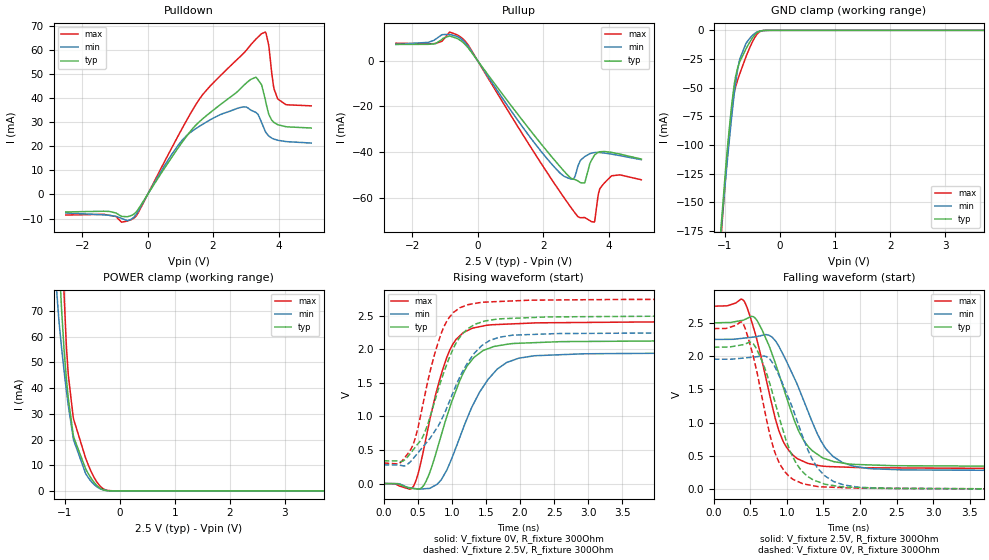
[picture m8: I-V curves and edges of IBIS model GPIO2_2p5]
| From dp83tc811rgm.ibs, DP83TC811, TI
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|   GPIO2_2p5 Model
[Model]   GPIO2_2p5
Model_type   I/O
Polarity   Non-Inverting
Enable   Active-Low
Vinl = 0.7
Vinh = 1.7
Vmeas = 1.25
Vref = 0
Cref = 2pF
Rref = 100000
|   typ   min   max
C_comp   3.2185pF   3.0315pF   3.3393pF
| Where Nom  PVT is Nominal Process, 2.5V, 27C
|   Fast PVT is Strong Process,  2.75V, -40C
|   Slow PVT is Weak Process,   2.25V, 125C
[Voltage Range]   2.5   2.25   2.75
|Junction Temperature
[Temperature Range]   27   125   -40
[Pullup Reference]   2.5   2.25   2.75
[Pulldown Reference]   0   0   0
[Power Clamp Reference]   2.5   2.25   2.75
[GND Clamp Reference]   0   0   0
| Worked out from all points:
|   slope of the pulldown table from 0 to 0.375 V, typ, clamps not added: 47.1 ohm
|   slope of the pullup table from 0 to 0.375 V, typ, clamps not added: 51.4 ohm
|   GND clamp passes 1 mA (typ) near -0.38 V on its own axis
|   POWER clamp passes 1 mA (typ) near -0.35 V on its own axis
|   falling waveform, V_fixture 2.5V, R_fixture 300Ohm: 20-80 % time 426ps typ, 473ps min, 334ps max; typ from 2.5 V to 0.339 V
|   rising waveform, V_fixture 0V, R_fixture 300Ohm: 20-80 % time 439ps typ, 535ps min, 364ps max; typ from 0 V to 2.13 V
|   rising waveform, V_fixture 2.5V, R_fixture 300Ohm: 20-80 % time 442ps typ, 590ps min, 359ps max; typ from 0.339 V to 2.5 V
|   falling waveform, V_fixture 0V, R_fixture 300Ohm: 20-80 % time 377ps typ, 428ps min, 307ps max; typ from 2.13 V to 0 V
[Pulldown]
|   Voltage   I(typ)   I(min)   I(max)
-2.5V     -7.255mA   -7.666mA   -8.536mA
-407.5mV  -8.044mA   -9.291mA   -9.718mA
747.5mV   15.65mA    16.84mA    19.61mA
1.34V     26.78mA    26.11mA    34.31mA
2.9V      44.79mA    36.31mA    58.19mA
3.312V    48.7mA     34.06mA    64.56mA
3.485V    45.46mA    29.83mA    66.8mA
3.62V     37.78mA    25.65mA    66.86mA
3.71V     33.06mA    24.21mA    61.1mA
3.845V    30.12mA    23.09mA    45.22mA
3.98V     28.98mA    22.52mA    39.66mA
5V        27.61mA    21.36mA    36.81mA
[GND Clamp]
|   Voltage   I(typ)   I(min)   I(max)
-2.5V     -1.255A    -1.134A    -1.35A
-1.067V   -171.4mA   -175.1mA   -180.1mA
-985mV    -120.8mA   -129.8mA   -127.2mA
-962.5mV  -108.2mA   -118.1mA   -113.7mA
-880mV    -67.32mA   -77.6mA    -70.77mA
-842.5mV  -52.25mA   -61.1mA    -57.64mA
-805mV    -40.55mA   -46.45mA   -49.4mA
-730mV    -27.57mA   -25.3mA    -38.07mA
-617.5mV  -16.29mA   -11.63mA   -23.27mA
-407.5mV  -1.86mA    -1.33mA    -3.018mA
-197.5mV  -14.99uA   -21.02uA   -19.14uA
5V        0A         0A         0A
[Pullup]
|   Voltage   I(typ)   I(min)   I(max)
-2.5V     7.194mA    7.203mA    7.713mA
-1.278V   7.641mA    9.595mA    7.627mA
-850mV    10.89mA    11.57mA    12.6mA
-437.5mV  7.916mA    8.747mA    9.422mA
2.397V    -44.38mA   -47.43mA   -54.94mA
2.915V    -51.88mA   -51.81mA   -65.59mA
3.065V    -52.69mA   -46.03mA   -68.29mA
3.268V    -53.51mA   -41.98mA   -68.7mA
3.56V     -41.53mA   -40.23mA   -70.73mA
3.695V    -40mA      -40.19mA   -57.87mA
4.1V      -40.17mA   -40.92mA   -50.36mA
5V        -43.06mA   -43.34mA   -52.15mA
[POWER Clamp]
|   Voltage   I(typ)   I(min)   I(max)
-2.5V     1.378A     1.128A     1.575A
-1.173V   138.2mA    86.25mA    204.3mA
-1.105V   95.25mA    67.15mA    145.5mA
-1.075V   79.94mA    60.23mA    121.4mA
-1.06V    73.26mA    56.99mA    110.2mA
-1.008V   54.58mA    46.52mA    75.98mA
-970mV    44.54mA    39.67mA    57.97mA
-932.5mV  36.21mA    33.3mA     45.26mA
-842.5mV  21.82mA    20.63mA    28.66mA
-617.5mV  8.611mA    6.772mA    12.78mA
-355mV    1.092mA    848.1uA    1.9mA
5V        0A         0A         0A
[Ramp]
R_load = 300
|   typ   min   max
dV/dt_r   1.27951/4.3828e-10   1.17145/5.33755e-10   1.44729/3.6279e-10
dV/dt_f   1.29582/4.22384e-10   1.1823/4.69132e-10   1.46485/3.31231e-10
[Falling Waveform]
V_fixture = 2.5V
V_fixture_min = 2.25V
V_fixture_max = 2.75V
R_fixture = 300Ohm
C_fixture = 0F
|   Time   V(typ)   V(min)   V(max)
0s        2.498V     2.249V     2.749V
419.9ps   2.546V     2.27V      2.815V
574.2ps   2.559V     2.289V     2.31V
800.6ps   2.02V      2.281V     1.245V
1.034ns   1.249V     1.828V     571mV
1.233ns   727mV      1.321V     413.3mV
1.464ns   488.1mV    726.4mV    349.6mV
1.761ns   392.8mV    400.5mV    332.7mV
2.586ns   351.9mV    289.5mV    318.7mV
20ns      338.8mV    278.7mV    307.4mV
[Rising Waveform]
V_fixture = 0V
V_fixture_min = 0V
V_fixture_max = 0V
R_fixture = 300Ohm
C_fixture = 0F
|   Time   V(typ)   V(min)   V(max)
0s        95.73uV    179.9uV    141.9uV
408.7ps   -70.99mV   -66mV      -75.15mV
583.6ps   -32.26mV   -77.9mV    491.2mV
769.5ps   459.9mV    -18.73mV   1.353V
972.7ps   1.141V     311.6mV    1.995V
1.221ns   1.745V     963.2mV    2.275V
1.506ns   2V         1.514V     2.357V
1.979ns   2.09V      1.867V     2.383V
2.927ns   2.117V     1.933V     2.4V
20ns      2.133V     1.953V     2.412V
[Rising Waveform]
V_fixture = 2.5V
V_fixture_min = 2.25V
V_fixture_max = 2.75V
R_fixture = 300Ohm
C_fixture = 0F
|   Time   V(typ)   V(min)   V(max)
0s        338.8mV    278.7mV    307.4mV
229ps     330.3mV    275.2mV    299.7mV
419.9ps   485.7mV    357.3mV    550.9mV
605.9ps   770.4mV    582.9mV    1.326V
791.5ps   1.37V      844.8mV    2.078V
933ps     1.797V     1.145V     2.434V
1.143ns   2.217V     1.643V     2.629V
1.414ns   2.398V     2.029V     2.697V
2.542ns   2.483V     2.234V     2.735V
20ns      2.498V     2.248V     2.748V
[Falling Waveform]
|Gnd
V_fixture = 0V
V_fixture_min = 0V
V_fixture_max = 0V
R_fixture = 300Ohm
C_fixture = 0F
|   Time   V(typ)   V(min)   V(max)
0s        2.133V     1.952V     2.412V
403.8ps   2.171V     1.97V      2.48V
542.4ps   2.181V     1.985V     1.985V
767.1ps   1.582V     1.953V     816.3mV
887.6ps   1.108V     1.718V     414.4mV
1.051ns   551.6mV    1.294V     175.9mV
1.414ns   117.2mV    326.1mV    40.48mV
1.781ns   32.95mV    62.78mV    22.67mV
2.461ns   12.45mV    9.693mV    11.83mV
20ns      95.29uV    188.6uV    140.8uV
